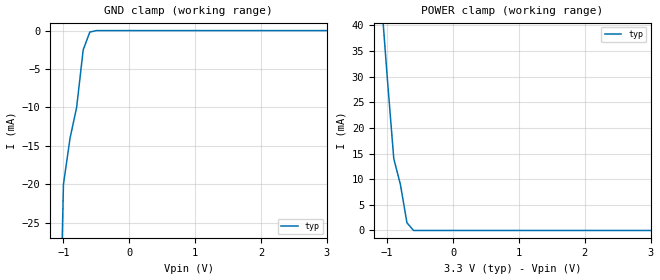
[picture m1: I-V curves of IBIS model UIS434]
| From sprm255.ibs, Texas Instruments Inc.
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[Model]   UIS434
Model_type   Input
Polarity   Non-Inverting
| signals   XI, CTRL, GZ, PWRDN, XOI, XIA, YI
Vinl = 0.8V
Vinh = 2.0V
|   typ   min   max
C_comp   2.2227p   2.2062p   2.2390p
|   typ   min   max
[Temperature Range]   25.0   -40   125
|   typ   min   max
[Voltage Range]   3.3V   3.0V   3.6V
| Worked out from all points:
|   GND clamp passes 1 mA (typ) near -0.63 V on its own axis
|   POWER clamp passes 1 mA (typ) near -0.67 V on its own axis
[GND_clamp]
|   Voltage   I(typ)   I(min)   I(max)
-3V       -900mA     NA         NA
-2V       -400mA     NA         NA
-1V       -20mA      NA         NA
-900mV    -14mA      NA         NA
-800mV    -10mA      NA         NA
-700mV    -2.5mA     NA         NA
-600mV    -200uA     NA         NA
-500mV    0A         NA         NA
3V        0A         NA         NA
[POWER_clamp]
|   Voltage   I(typ)   I(min)   I(max)
-3V       600mA      NA         NA
-2V       200mA      NA         NA
-1V       30mA       NA         NA
-900mV    14mA       NA         NA
-800mV    9mA        NA         NA
-700mV    1.5mA      NA         NA
-600mV    0A         NA         NA
-500mV    0A         NA         NA
3V        0A         NA         NA
